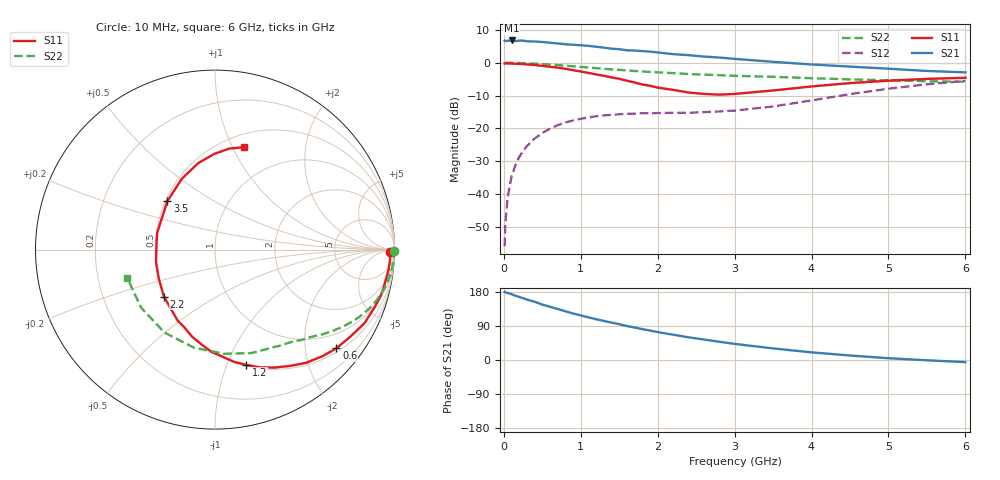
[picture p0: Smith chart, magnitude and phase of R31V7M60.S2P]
! SIEMENS Small Signal Semiconductors
! BFR181
! Si NPN RF Bipolar Junction Transistor in SOT23
! VCE = 1.75 V  IC = 0.6 mA
! Common Emitter S-Parameters:  May  1996
# GHz  S  MA  R  50
!  f  S11  S21  S12  S22
! GHz  MAG  ANG  MAG  ANG  MAG  ANG  MAG  ANG
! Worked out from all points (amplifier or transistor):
!   36 points, 10 MHz to 6 GHz, reference 50 ohm
!   highest |S21| = 6.8 dB at 100 MHz (marker M1)
!   |S21| within 3 dB of that: start of sweep to 1.601 GHz
!   unconditionally stable (mu >= 1): 2.253 GHz to 3.95 GHz
!   at 250 MHz: K = 0.13, MSG = 16.8 dB, |S12| = -26.9 dB
!   at 1.4 GHz: K = 0.66, MSG = 10.1 dB, |S12| = -15.9 dB
!   at 6 GHz: K = 0.92, MSG = 1.3 dB, |S12| = -5.5 dB
!   S11 on the Smith chart (normalised r, x): 10 MHz: 68, -36; 600 MHz: 0.59, -2.70; 1.2 GHz: 0.51, -1.17; 2.2 GHz: 0.49, -0.30; 3.5 GHz: 0.51, +0.32; 6 GHz: 0.63, +1.10
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0.01  0.9774 -0.7  2.182 179.8  0.0016 93.2  0.9995 -0.3
0.02  0.9763 -1.2  2.138 178.5  0.0036 82.7  0.9929 -0.6
0.05  0.9771 -3.3  2.167 176.9  0.0089 87.3  0.9994 -1.6
0.1  0.9731 -6.8  2.192 173.7  0.0185 85.0  0.9976 -3.1
0.15  0.9665 -9.9  2.145 169.6  0.0273 82.9  0.9937 -4.7
0.2  0.9631 -13.2  2.175 166.4  0.0367 81.0  0.9907 -6.3
0.3  0.9456 -19.8  2.13 159.5  0.0536 76.4  0.982 -9.4
0.4  0.9284 -26.2  2.113 153.7  0.0699 72.2  0.9719 -12.3
0.5  0.8965 -32.7  2.078 146.2  0.085 68.1  0.9565 -15.2
0.6  0.8718 -39.1  2.024 140.5  0.0992 64.1  0.9398 -18.0
0.9  0.7735 -56.8  1.885 122.7  0.1325 53.5  0.8857 -25.2
1.1  0.7018 -69.2  1.814 112.6  0.1471 47.9  0.8471 -29.4
1.2  0.6648 -74.9  1.76 107.6  0.1532 45.1  0.8292 -31.5
1.6  0.533 -98.2  1.552 89.6  0.1669 38.1  0.7672 -37.8
1.9  0.4467 -117.9  1.481 77.7  0.1701 36.0  0.7251 -42.1
2.2  0.3868 -137.4  1.356 66.8  0.1725 35.2  0.696 -46.4
2.4  0.3523 -152.8  1.308 59.9  0.1729 36.5  0.6746 -49.2
2.8  0.3268 177.0  1.203 48.2  0.1812 40.0  0.6477 -55.6
3.5  0.3786 134.5  1.035 30.6  0.216 47.1  0.6116 -70.4
4.5  0.4904 101.1  0.875 11.9  0.333 47.7  0.5589 -102.1
5.5  0.5689 81.9  0.751 -0.7  0.4703 35.1  0.5237 -141.9
6  0.5915 74.4  0.715 -5.6  0.5297 26.7  0.5137 -162.2
